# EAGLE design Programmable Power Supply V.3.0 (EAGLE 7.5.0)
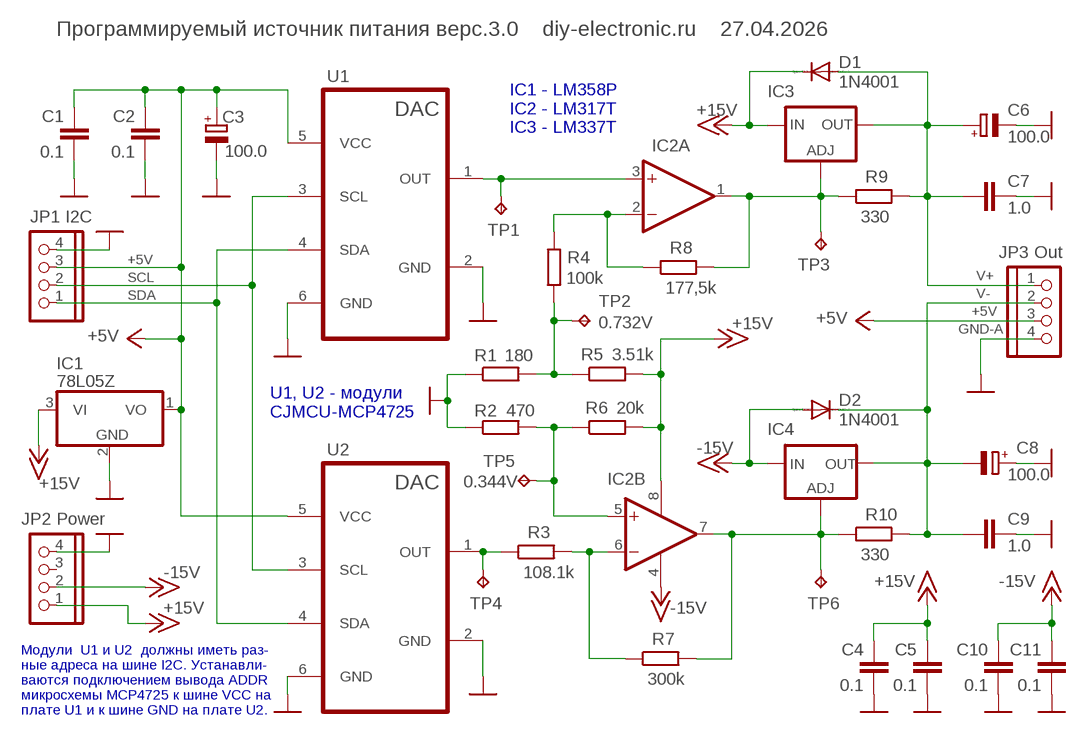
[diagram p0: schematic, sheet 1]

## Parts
C1  0.1  C-EU050-025X075  [C050-025X075]
C2  0.1  C-EU050-025X075  [C050-025X075]
C3  100.0  CPOL-EUE2.5-7  [E2,5-7]
C4  0.1  C-EU050-025X075  [C050-025X075]
C5  0.1  C-EU050-025X075  [C050-025X075]
C6  100.0  CPOL-EUE2.5-7  [E2,5-7]
C7  1.0  C-EU050-025X075  [C050-025X075]
C8  100.0  CPOL-EUE2.5-7  [E2,5-7]
C9  1.0  C-EU050-025X075  [C050-025X075]
C10  0.1  C-EU050-025X075  [C050-025X075]
C11  0.1  C-EU050-025X075  [C050-025X075]
D1  1N4001  DIODE-DO41-7.6  [DO41-7.6]
D2  1N4001  DIODE-DO41-7.6  [DO41-7.6]
IC1  78L05Z  [TO92]
IC2  LM358N  [DIL08]
IC3  LM317T  LM317TS  [317TS]
IC4  LM337T  LM337TS  [337TS]
JP1  I2C  PINHD-1X4  [1X04]
JP2  Power  PINHD-1X4  [1X04]
JP3  Out  PINHD-1X4  [1X04]
R1  180  R-EU_0204/7  [0204/7]
R2  470  R-EU_0207/10  [0207/10]
R3  108.1k  R-EU_0204/7  [0204/7]
R4  100k  R-EU_0204/7  [0204/7]
R5  3.51k  R-EU_0204/7  [0204/7]
R6  20k  R-EU_0204/7  [0204/7]
R7  300k  R-EU_0204/7  [0204/7]
R8  177,5k  R-EU_0204/7  [0204/7]
R9  330  R-EU_0204/7  [0204/7]
R10  330  R-EU_0204/7  [0204/7]
TP1  TPPAD1-13  [P1-13]
TP2  TPPAD1-13  [P1-13]
TP3  TPPAD1-13  [P1-13]
TP4  TPPAD1-13  [P1-13]
TP5  TPPAD1-13  [P1-13]
TP6  TPPAD1-13  [P1-13]
U1  MCP4725-MODULE  [6-PIN-MODULE-4725]
U2  MCP4725-MODULE  [6-PIN-MODULE-4725]

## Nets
+5V: C1.2 C2.2 C3.+ IC1.1(VO) JP1.3 JP3.3 U1.5(VCC) U2.5(VCC)
+15V: C4.2 C5.2 D1.C IC1.3(VI) IC2.8(P:V+) IC3.3(IN) JP2.1 R5.2 R6.2
-15V: C10.2 C11.2 D2.A IC2.4(P:V-) IC4.2(IN) JP2.2
GND-A: C1.1 C2.1 C3.- C4.1 C5.1 C6.- C7.1 C8.+ C9.1 C10.1 C11.1 IC1.2(GND) JP1.4 JP2.4 JP3.4 R1.1 R2.1 U1.2(GND) U1.6(GND) U2.2(GND) U2.6(GND) ; supply symbol labelled GND
N$1: IC2.3(A:+IN) TP1.TP U1.1(OUT)
N$2: IC2.2(A:-IN) R4.2 R8.1
N$3: R3.1 TP4.TP U2.1(OUT)
N$4: IC2.1(A:OUT) IC3.1(ADJ) R8.2 R9.1 TP3.TP
N$9: IC2.6(B:-IN) R3.2 R7.1
N$10: IC2.7(B:OUT) IC4.1(ADJ) R7.2 R10.1 TP6.TP
N$12: R1.2 R4.1 R5.1 TP2.TP
N$13: IC2.5(B:+IN) R2.2 R6.1 TP5.TP
SCL: JP1.2 U1.3(SCL) U2.3(SCL)
SDA: JP1.1 U1.4(SDA) U2.4(SDA)
V+: C6.+ C7.2 D1.A IC3.2(OUT) JP3.1 R9.2
V-: C8.- C9.2 D2.C IC4.3(OUT) JP3.2 R10.2
Unconnected: JP2.3

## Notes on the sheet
- Программируемый источник питания верс.3.0    diy-electronic.ru    27.04.2026
- IC1 - LM358P
  IC2 - LM317T
  IC3 - LM337T
- +5V
- SCL | V+
- SDA | V-
- +5V
- GND-A
- U1, U2 - модули 
  CJMCU-MCP4725
- Модули  U1 и U2  должны иметь раз- 
  ные адреса на шине I2C. Устанавли-
  ваются подключением вывода ADDR
  микросхемы MCP4725 к шине VCC на
  плате U1 и к шине GND на плате U2.

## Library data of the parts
C1 C2 C4 C5 C7 C9-C11 = resistor:C-EU: CAPACITOR, European symbol
C3 C6 C8 = resistor:CPOL-EU: POLARIZED CAPACITOR, European symbol
D1 D2 = diode:DIODE-: DIODE
IC1 = linear:78*: Positive VOLTAGE REGULATOR Source: http://cache.national.com/ds/LM/LM78L05.pdf http://www.fairchildsemi.com/ds/LM/LM7805.pdf
IC2 = linear:LM358: OP AMP also LM158; LM258; LM2904 Source: http://cache.national.com/ds/LM/LM158.pdf
IC3 = v-reg:LM317TS: VOLTAGE REGULATOR
IC4 = v-reg:LM337TS: VOLTAGE REGULATOR
JP1-JP3 = pinhead:PINHD-1X4: PIN HEADER
R1-R10 = resistor:R-EU_: RESISTOR, European symbol
TP1 TP3 TP4 TP6 = testpad:TP: Test pad
TP2 = testpad:TP: Test pad; TP_SIGNAL_NAME: 0.732V
TP5 = testpad:TP: Test pad; TP_SIGNAL_NAME: 0.344V
U1 U2 = FRMeterCustomComponents:MCP4725-MODULE: 12-bit DAC module based on MCP4725

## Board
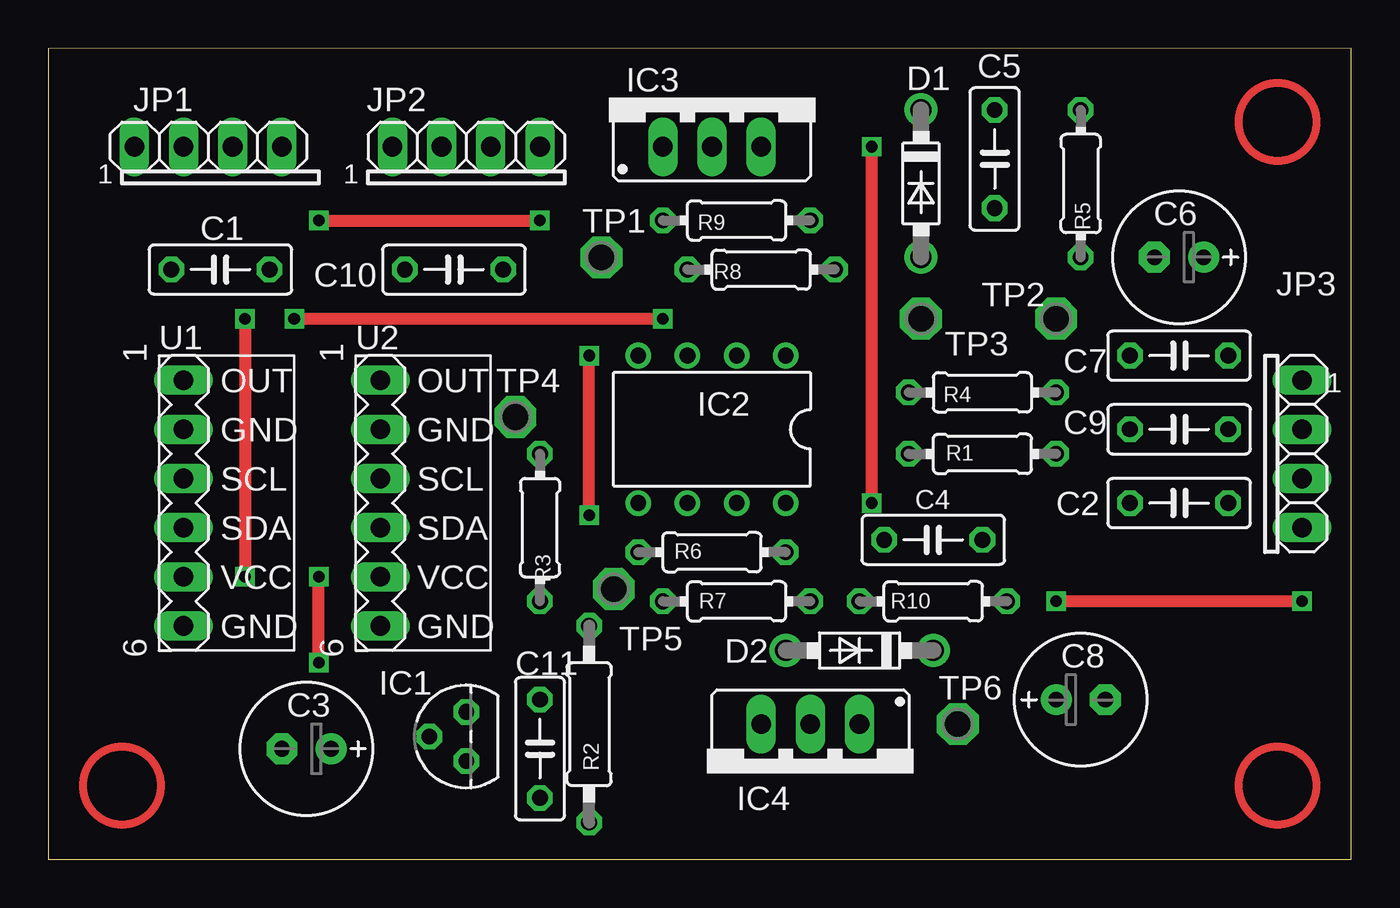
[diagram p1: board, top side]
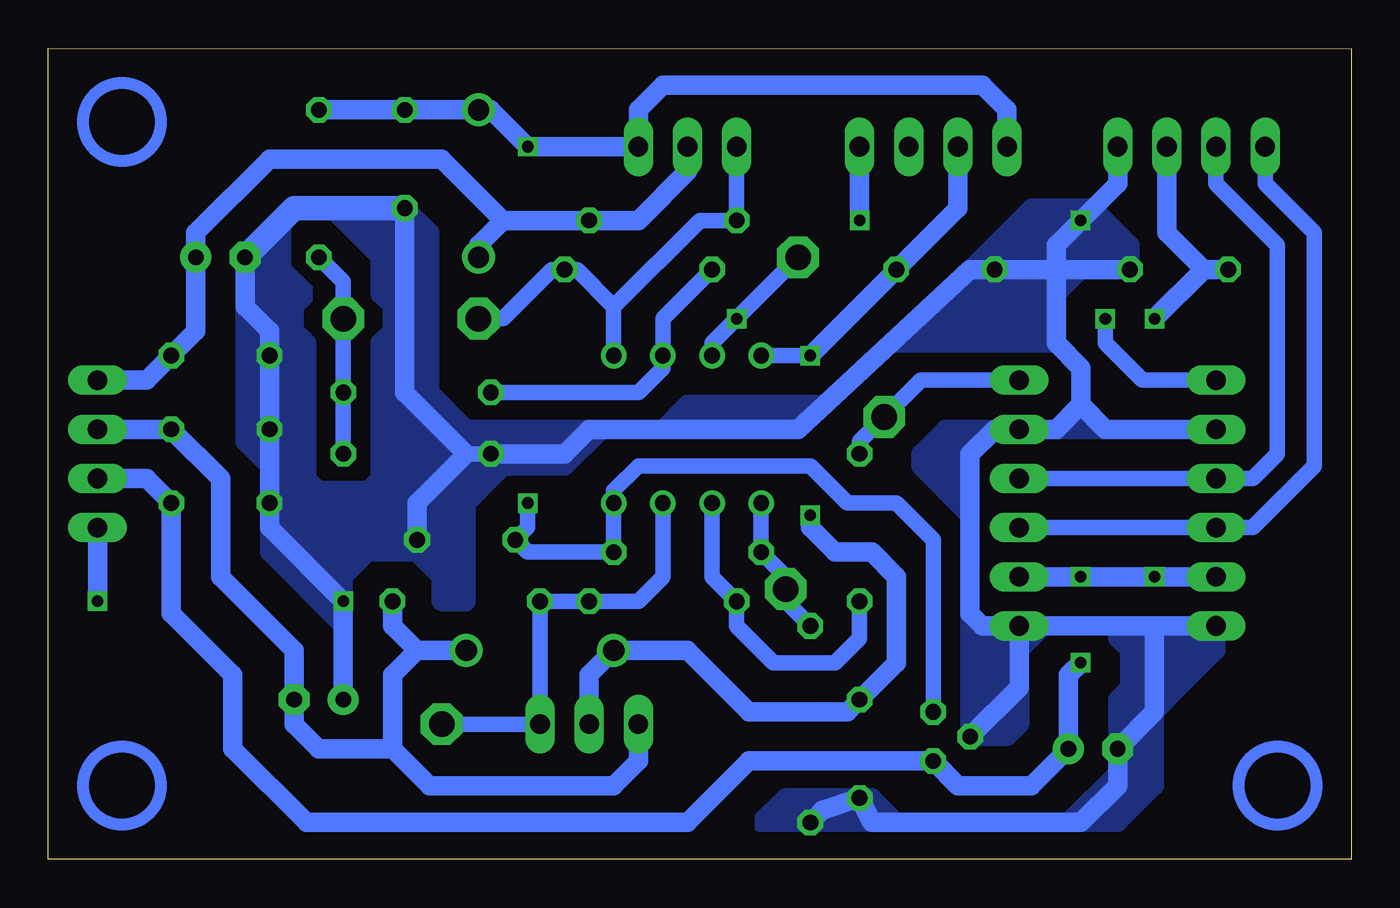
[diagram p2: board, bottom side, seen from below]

Size 67.31 x 41.91 mm. Coordinates in mm from the lower left corner, seen from the top.
Outline: 0,0 67.31,0 67.31,41.91 0,41.9 0,0
Copper layers (1*16): Top 0.035mm / dielectric 1.5mm / Bottom 0.035mm
Design rules "default *": minimum track width 10mil, minimum drill 10mil, track to track 16mil, track to pad 16mil, pad to pad 8mil, via to via 8mil, smd to smd 8mil, copper to edge 1mil, drill to drill 8mil, minimum pad ring 10mil, minimum via ring 8mil, stop-mask expansion 4mil, vias tented up to drill 0mil, thermal gap 10mil

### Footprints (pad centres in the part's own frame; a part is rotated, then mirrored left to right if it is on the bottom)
C050-025X075 = drill 0.813 octagon: 1 -2.54,0; 2 2.54,0
E2,5-7 = drill 0.813 pad 1.6: + -1.27,0 | drill 0.813 pad 1.6 octagon: - 1.27,0
DO41-7.6 = drill 1.1 pad 1.7: A 3.81,0; C -3.81,0
TO92 = drill 0.813 octagon: 1 -1.27,0; 2 0,1.905; 3 1.27,0
DIL08 = drill 0.813 pad 1.27: 1 -3.81,-3.81; 2 -1.27,-3.81; 3 1.27,-3.81; 4 3.81,-3.81; 5 3.81,3.81; 6 1.27,3.81; 7 -1.27,3.81; 8 -3.81,3.81
317TS = drill 1.016 long: 1 -2.54,-2.54; 2 0,-2.54; 3 2.54,-2.54
337TS = drill 1.016 long: 1 -2.54,-2.54; 2 0,-2.54; 3 2.54,-2.54
1X04 = drill 1.016 long: 1 -3.81,0; 2 -1.27,0; 3 1.27,0; 4 3.81,0
0204/7 = drill 0.813 octagon: 1 -3.81,0; 2 3.81,0
0207/10 = drill 0.813 octagon: 1 -5.08,0; 2 5.08,0
P1-13 = drill 1.321 pad 2.159 octagon: TP 0,0
6-PIN-MODULE-4725 = drill 1.016 long: 1 -6.35,-2.54; 2 -3.81,-2.54; 3 -1.27,-2.54; 4 1.27,-2.54; 5 3.81,-2.54; 6 6.35,-2.54

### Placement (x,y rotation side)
C1  8.89,30.48 180 top
C2  58.42,18.41 0 top
C3  13.33,5.71 180 top
C4  45.72,16.51 180 top
C5  48.9,36.2 90 top
C6  58.42,31.11 180 top
C7  58.42,26.04 0 top
C8  53.34,8.26 0 top
C9  58.42,22.22 0 top
C10  20.95,30.48 0 top
C11  25.4,5.71 90 top
D1  45.09,34.93 270 top
D2  41.91,10.79 180 top
IC1  21.59,6.35 90 top
IC2  34.29,22.22 180 top
IC3  34.29,39.37 0 top
IC4  39.37,4.45 180 top
JP1  8.26,36.83 0 top
JP2  21.59,36.83 0 top
JP3  64.77,20.95 270 top
R1  48.26,20.95 0 top
R2  27.94,6.98 90 top
R3  25.4,17.14 270 top
R4  48.26,24.13 180 top
R5  53.34,34.93 90 top
R6  34.29,15.88 0 top
R7  35.56,13.33 0 top
R8  36.83,30.48 0 top
R9  35.56,33.02 0 top
R10  45.72,13.33 0 top
TP1  28.57,31.11 0 top
TP2  52.07,27.94 0 top
TP3  45.09,27.94 0 top
TP4  24.13,22.86 0 top
TP5  29.21,13.97 0 top
TP6  46.99,6.98 0 top
U1  9.53,18.41 270 top
U2  19.68,18.41 270 top

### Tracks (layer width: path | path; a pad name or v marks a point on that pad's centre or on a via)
+5V  (via drill 0.6)
  Top 0.61: v10.16,27.94 v10.16,14.61 | v13.97,10.16 v13.97,14.61
  Bottom 1.016: JP3.3 62.23,19.68 C2.2 60.96,12.7 57.79,9.53 57.79,5.71 53.98,1.91 34.29,1.91 31.11,5.08 IC1.1 20.32,3.81 16.51,3.81 C3.+ 14.61,9.53 v13.97,10.16 | 7.62,30.48 9.53,32.38 JP1.3 | 7.62,30.48 v10.16,27.94 | U1.5 v10.16,14.61 v13.97,14.61 U2.5 | C1.2 7.62,30.48
+15V  (via drill 0.6)
  Top 0.61: v42.55,18.41 v42.55,36.83
  Bottom 0.813: v42.55,18.41 42.55,17.14 C4.2 42.55,15.88 R6.2 IC2.8 38.1,19.05 36.83,20.32 27.94,20.32 26.04,18.41 23.5,18.41 21.59,16.51 IC1.3 | D1.C 44.45,38.74
  Bottom 1.016: 44.45,38.74 v42.55,36.83 IC3.3 36.83,38.74 35.56,40.01 19.05,40.01 17.78,38.74 JP2.1 | D1.C C5.2 R5.2
-15V  (via drill 0.6)
  Top 0.61: v27.94,17.78 v27.94,26.04
  Bottom 0.813: v27.94,26.04 IC2.4
  Bottom 1.016: IC4.2 39.37,9.53 D2.A 34.29,10.79 31.11,7.62 26.04,7.62 C11.2 23.5,10.16 23.5,14.61 24.77,15.88 26.67,15.88 27.94,17.14 v27.94,17.78 | v27.94,26.04 C10.2 20.32,33.66 JP2.2
GND-A  (via drill 0.6)
  Top 0.61: v13.97,33.02 v25.4,33.02 | v64.77,13.33 v52.07,13.33
  Bottom 0.813: R1.1 45.72,20.95
  Bottom 1.016: 15.24,30.48 15.24,31.75 v13.97,33.02 12.06,34.93 JP1.4 | v25.4,33.02 JP2.4 | 15.24,30.48 C10.1 19.68,30.48 28.57,22.22 39.37,22.22 40.64,20.95 R1.1 | 15.24,30.48 C1.1 | U1.6 10.16,12.06 | 10.16,12.06 U2.6 | U1.2 12.7,22.22 13.97,23.5 | 13.97,23.5 15.24,22.22 U2.2 18.41,22.22 19.68,20.95 19.68,12.7 19.05,12.06 U2.6 | 13.97,23.5 13.97,25.4 15.24,26.67 15.24,30.48 | 10.16,12.06 10.16,7.62 C3.- 12.06,3.81 13.97,1.91 24.77,1.91 C11.1 27.3,2.54 R2.1 | C5.1 48.9,24.13 45.72,20.95 48.26,18.41 C4.1 | C6.- 57.15,28.57 55.88,27.3 C7.1 C9.1 C2.1 55.88,17.14 v52.07,13.33 C8.+ | JP3.4 v64.77,13.33 | IC1.2 17.14,8.89 U2.6
  Bottom 1.27: C5.1 54.61,33.66 C6.-
  pour Bottom (no thermals): 48.9,33.66 52.71,33.66 50.17,31.11 50.17,29.21 49.53,28.57 49.53,27.3 50.17,26.67 50.17,19.68 50.8,19.05 53.34,19.05 53.34,17.78 52.07,15.88 46.36,15.88 45.72,17.14 45.72,22.22 47.62,24.13 47.62,32.38
  pour Bottom (no thermals): 53.34,19.05 53.98,19.68 53.98,26.67 54.61,27.3 54.61,28.57 53.98,29.21 55.25,30.48 55.25,33.02 57.15,31.11 57.15,21.59 55.88,20.32 55.88,15.88 52.07,12.06 52.07,14.61 47.62,19.05
  pour Bottom (no thermals): 15.24,26.67 23.5,26.67 16.51,33.66 13.33,33.66 11.43,31.75 11.43,30.48 13.97,30.48 15.24,29.21
  pour Bottom (no thermals): 46.36,22.86 43.82,20.32 46.36,17.78
  pour Bottom (no thermals): 27.3,23.5 34.29,23.5 35.56,22.22 28.57,22.22
  pour Bottom (no thermals): 38.74,22.22 40.64,20.32 46.36,20.32 46.36,22.22
  pour Bottom (no thermals): 19.68,6.35 19.68,12.7 19.05,12.06 15.88,12.06 17.14,10.79 17.14,6.98 17.78,6.35
  pour Bottom (no thermals): 18.41,22.22 20.95,22.22 22.22,20.95 22.22,20.32 19.68,17.78 19.68,20.95
  pour Bottom (no thermals): 12.06,5.71 6.98,10.79 6.98,12.06 12.06,12.06 12.06,11.43 11.43,10.79 11.43,8.89 12.06,8.26
  pour Bottom (no thermals): 48.9,16.51 46.99,14.61 46.99,13.33 45.72,13.33 45.72,19.68 48.9,19.68
  pour Bottom (no thermals): 10.16,7.62 10.16,3.81 12.06,1.91 14.61,1.91 12.06,4.45 12.06,6.98 11.43,7.62
  pour Bottom (no thermals): 23.5,1.91 24.77,3.17 29.21,3.17 30.48,1.91
  pour Bottom (no thermals): 13.97,23.5 12.7,22.22 15.24,22.22
N$1  (via drill 0.6)
  Top 0.61: v12.7,27.94 v31.75,27.94
  Bottom 0.813: U1.1 10.79,24.77 12.7,26.67 v12.7,27.94 | IC2.3 33.02,26.67 v31.75,27.94 TP1.TP
N$2
  Bottom 0.813: R8.1 35.56,27.94 IC2.2 35.56,25.4 36.83,24.13 R4.2
N$3
  Bottom 0.813: U2.1 22.22,24.77 TP4.TP 25.4,21.59 R3.1
N$4
  Bottom 0.813: IC3.1 R9.1 33.66,33.02 38.1,28.57 | 38.1,28.57 IC2.1 | 38.1,28.57 40.01,30.48 R8.2 41.28,30.48 43.82,27.94 TP3.TP
N$9
  Bottom 0.813: R3.2 25.4,11.43 26.67,10.16 29.84,10.16 31.75,12.06 R7.1 33.02,14.61 IC2.6
N$10
  Bottom 0.813: IC2.7 35.56,14.61 36.83,13.33 R7.2 R10.1 IC4.1 TP6.TP
N$12
  Bottom 0.813: R5.1 52.07,29.84 TP2.TP R4.1 R1.2
N$13
  Bottom 0.813: IC2.5 R6.1 29.21,14.61 TP5.TP 29.21,13.33 R2.2
SCL
  Bottom 0.813: U2.3 U1.3 5.08,19.68 3.81,20.95 3.81,31.75 6.98,34.93 JP1.2
SDA
  Bottom 0.813: U2.4 U1.4 5.08,17.14 1.91,20.32 1.91,32.38 4.45,34.93 JP1.1
V+
  Bottom 1.016: D1.A 45.09,31.75 43.82,33.02 | IC3.2 34.29,35.56 36.83,33.02 R9.2 43.82,33.02 | JP3.1 62.23,24.77 C7.2 59.69,27.3 C6.+ 59.69,32.38 55.88,36.2 46.99,36.2 43.82,33.02
V-
  Bottom 1.016: JP3.2 C9.2 58.42,19.68 58.42,14.61 54.61,10.79 C8.- 54.61,6.98 53.34,5.71 49.53,5.71 | IC4.3 36.83,5.08 38.1,3.81 47.62,3.81 49.53,5.71 | 48.26,10.79 D2.C | 48.26,10.79 49.53,12.06 R10.2 | 48.26,10.79 49.53,9.53 49.53,5.71
(copper drawn outside any net)
  shapes: Bottom circle x3, Top circle x3

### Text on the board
tPlace: 1 | 1 | 1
